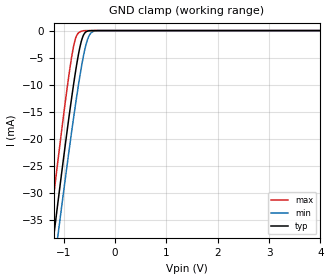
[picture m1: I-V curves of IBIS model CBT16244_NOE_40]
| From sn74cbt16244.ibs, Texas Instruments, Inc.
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[Model]   CBT16244_NOE_40
Model_type  Input
Vinl = 0.8
Vinh = 2.0
| variable   typ   min   max
C_comp   1.41pF   1.13pF   1.76pF
[Temperature Range]   40   100   -40
| Ambient temperature   25   85   -40
[Voltage range]   4   4   4
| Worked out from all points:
|   GND clamp passes 1 mA (typ) near -0.62 V on its own axis
[GND Clamp]
| CBT16244_NOE_40
|   Voltage   I(typ)   I(min)   I(max)
-4V       -265.8mA   -266.6mA   -266.2mA
-1.295V   -45.55mA   -51.37mA   -38.3mA
-1.26V    -42.84mA   -48.72mA   -35.49mA
-1.19V    -37.45mA   -43.46mA   -29.92mA
-1.105V   -31mA      -37.13mA   -23.27mA
-945mV    -19.21mA   -25.5mA    -11.31mA
-830mV    -11.28mA   -17.5mA    -3.946mA
-760mV    -6.903mA   -12.88mA   -1.15mA
-675mV    -2.605mA   -7.728mA   -192.1uA
-535mV    -90.35uA   -1.582mA   -297.4nA
-390mV    -1.069uA   -63.5uA    -872.3pA
4V        33.47pA    2.709nA    26.57pA
